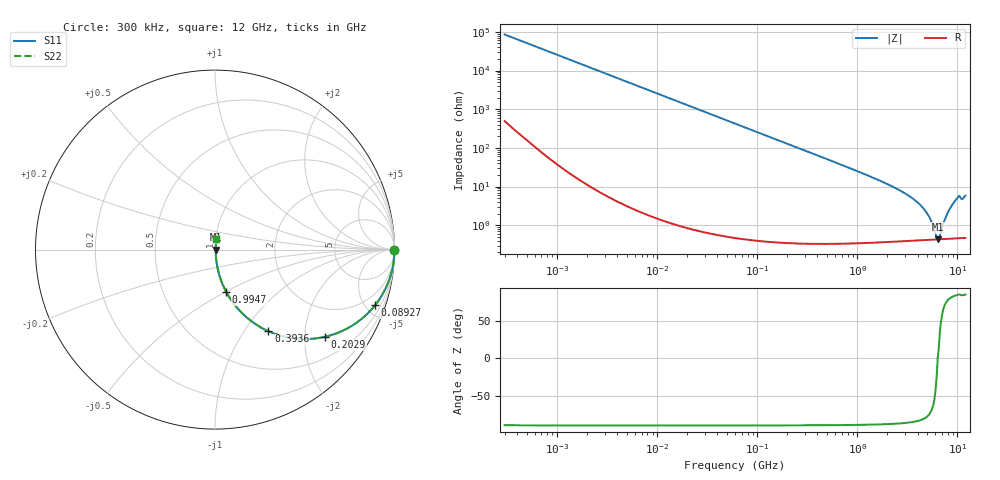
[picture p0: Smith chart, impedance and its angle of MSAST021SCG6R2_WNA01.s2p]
! MSAST021SCG6R2_WNA01  S-PARAMETER MODEL  ( General Type )
! Model Generated by TAIYO YUDEN Corporation (http://www.ty-top.com)
! Version 2.0
! TAIYO YUDEN Control No. 181101
! Copyright(c) 2015 TAIYO YUDEN CO.,LTD. All Rights Reserved.
! Product Description (link to TY-COMPAS)
! https://ds.yuden.co.jp/TYCOMPAS/or/detail?pn=MSAST021SCG6R2CWNA01&u=M
! Products Name : Multilayer Ceramic Capacitors
! Characteristics :
!  Capacitance : 6.2 pF , Rated Voltage : 25V , TCC : CG / C0G
!  Case Size : 0.25 x 0.125 / 0.0098 x 0.0049 [mm/inch] , Thickness : 0.125 / 0.0049 [mm/inch]
!  (Conditions: Temperature = 25 degC , DC Bias Current/Voltage = 0A / 0V)
! External Node Assignments :
!  1  o---| |---o  2
! GND o---------o GND
! Frequency Range : 0.3MHz  -  12000MHz  [ 401 STEP ]
# MHz S RI R 50
! Freq[MHz].  S11 Real  S11 Imag  S21 Real  S21 Imag  S12 Real  S12 Imag  S22 Real  S22 Imag
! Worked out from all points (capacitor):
!   401 points, 300 kHz to 12 GHz, reference 50 ohm
!   read as one part in series: C = 6.2 pF near 316.3 kHz
!   lowest |Z| = 434 mohm at 6.354 GHz (marker M1)
!   series resonance near 6.35 GHz, so ESL is about 100 pH
!   S11 on the Smith chart (normalised r, x): 300 kHz: open; 89.27 MHz: 1.01, -5.75; 202.9 MHz: 1.01, -2.53; 393.6 MHz: 1.01, -1.30; 994.7 MHz: 1.01, -0.50; 12 GHz: 1.01, +0.12
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0.3  1 -0.00117  8.09e-06 0.00117  8.09e-06 0.00117  1 -0.00117
1.769972  0.9999 -0.00689  5.4e-05 0.00689  5.4e-05 0.00689  0.9999 -0.00689
10.44266  0.9983 -0.0406  0.00168 0.0406  0.00168 0.0406  0.9983 -0.0406
27.82928  0.9883 -0.1071  0.0117 0.1071  0.0117 0.1071  0.9883 -0.1071
60  0.948 -0.2215  0.052 0.2215  0.052 0.2215  0.948 -0.2215
89.27472  0.8917 -0.31  0.1083 0.31  0.1083 0.31  0.8917 -0.31
202.9496  0.6146 -0.4853  0.3854 0.4853  0.3854 0.4853  0.6146 -0.4853
353.9943  0.3439 -0.4727  0.6561 0.4727  0.6561 0.4727  0.3439 -0.4727
393.5654  0.2978 -0.4548  0.7022 0.4548  0.7022 0.4548  0.2978 -0.4548
617.4538  0.147 -0.3501  0.853 0.3501  0.853 0.3501  0.147 -0.3501
994.7115  0.0624 -0.2352  0.9376 0.2352  0.9376 0.2352  0.0624 -0.2352
2088.533  0.0154 -0.1075  0.9846 0.1075  0.9846 0.1075  0.0154 -0.1075
3276.641  0.00719 -0.0568  0.9928 0.0568  0.9928 0.0568  0.00719 -0.0568
4385.161  0.00502 -0.0303  0.995 0.0303  0.995 0.0303  0.00502 -0.0303
5140.631  0.00449 -0.017  0.9955 0.017  0.9955 0.017  0.00449 -0.017
6026.253  0.00431 -0.00418  0.9957 0.00418  0.9957 0.00418  0.00431 -0.00418
6354.153  0.00432 4.75e-05  0.9957 -4.75e-05  0.9957 -4.75e-05  0.00432 4.75e-05
6699.894  0.00436 0.00348  0.9956 -0.00348  0.9956 -0.00348  0.00436 0.00348
7648.807  0.00467 0.0154  0.9953 -0.0154  0.9953 -0.0154  0.00467 0.0154
8966.534  0.00572 0.0345  0.9943 -0.0345  0.9943 -0.0345  0.00572 0.0345
9968.853  0.00703 0.0493  0.993 -0.0493  0.993 -0.0493  0.00703 0.0493
12000  0.00802 0.0574  0.992 -0.0574  0.992 -0.0574  0.00802 0.0574
